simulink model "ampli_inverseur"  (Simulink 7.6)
settings: Solver=ode15s  StartTime=0.0  StopTime=0.001  FixedStep=0.01  RelTol=1e-5
InitFcn:
  | clc
StopFcn:
  | % lecture du fichier binaire
  | load inverseur.mat
  | 
  | % trace de la tension et du courant d’induit
  | plot(x(1,:),x(2,:),x(1,:),x(3,:))
  | title('Entrée/sortie - amplificateur inverseur - Composant ampli op')
  | grid
libraries: fl_lib x11, nesl_utility x4, MaLibrairieElectrical_lib x1

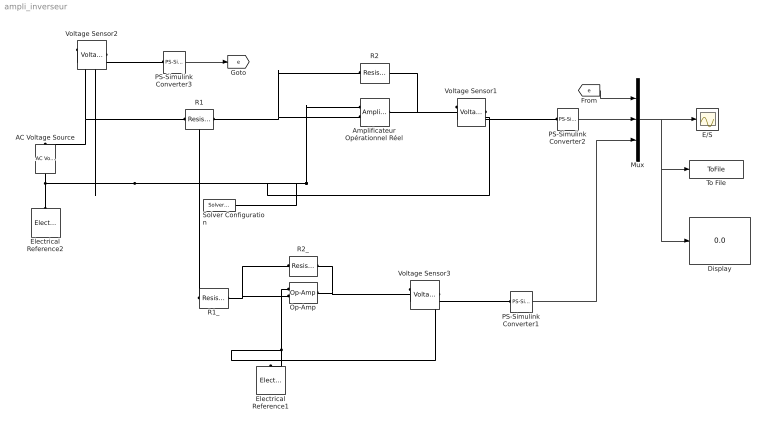
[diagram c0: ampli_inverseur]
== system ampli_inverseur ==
  AC Voltage Source : fl_lib/Electrical/Electrical Sources/AC Voltage Source  DialogController=NetworkEngine.DynNeDlgSource  SystemSampleTime=-1  amp=5 V  shift=0 rad  omega=2 kHz  i_Log=off  v_Log=off  LocalVarNames=|i|v  LocalVarDescs=|i|v  LocalVarLogging=[0 0]
  Amplificateur Opérationnel Réel : MaLibrairieElectrical_lib/Amplificateur Opérationnel Réel  DialogController=NetworkEngine.DynNeDlgSource  SystemSampleTime=-1  A=1e+6  Re=1e+6 Ohm  Rs=100 Ohm  Vsat=15 V  ie_Log=off  eps_Log=off  is_Log=off  vs_Log=off  LocalVarNames=|ie|eps|is|vs  LocalVarDescs=|ie|eps|is|vs  LocalVarLogging=[0 0 0 0]
  Display : Display
  E/S : Scope
  Electrical Reference1 : fl_lib/Electrical/Electrical Elements/Electrical Reference  DialogController=NetworkEngine.DynNeDlgSource  SystemSampleTime=-1  i_Log=off  LocalVarNames=|i  LocalVarDescs=|i  LocalVarLogging=0
  Electrical Reference2 : fl_lib/Electrical/Electrical Elements/Electrical Reference  DialogController=NetworkEngine.DynNeDlgSource  SystemSampleTime=-1  i_Log=off  LocalVarNames=|i  LocalVarDescs=|i  LocalVarLogging=0
  Mux : Mux  Inputs=3
  Op-Amp : fl_lib/Electrical/Electrical Elements/Op-Amp  DialogController=NetworkEngine.DynNeDlgSource  SystemSampleTime=-1  i1_Log=off  v1_Log=off  outI_Log=off  LocalVarNames=|i1|v1|outI  LocalVarDescs=|i1|v1|outI  LocalVarLogging=[0 0 0]
  PS-Simulink Converter1 : nesl_utility/PS-Simulink Converter  DialogController=NetworkEngine.DynNeUtilDlgSource  SystemSampleTime=-1  PhysicalDomain=network_engine_domain  LeftPortType=input  RightPortType=output  SubClassName=ps_output  Unit=1  AffineConversion=off
  PS-Simulink Converter2 : nesl_utility/PS-Simulink Converter  DialogController=NetworkEngine.DynNeUtilDlgSource  SystemSampleTime=-1  PhysicalDomain=network_engine_domain  LeftPortType=input  RightPortType=output  SubClassName=ps_output  Unit=1  AffineConversion=off
  PS-Simulink Converter3 : nesl_utility/PS-Simulink Converter  DialogController=NetworkEngine.DynNeUtilDlgSource  SystemSampleTime=-1  PhysicalDomain=network_engine_domain  LeftPortType=input  RightPortType=output  SubClassName=ps_output  Unit=1  AffineConversion=off
  R1 : fl_lib/Electrical/Electrical Elements/Resistor  DialogController=NetworkEngine.DynNeDlgSource  SystemSampleTime=-1  R=47 kOhm  i_Log=off  v_Log=off  LocalVarNames=|i|v  LocalVarDescs=|i|v  LocalVarLogging=[0 0]
  R1_ : fl_lib/Electrical/Electrical Elements/Resistor  DialogController=NetworkEngine.DynNeDlgSource  SystemSampleTime=-1  R=47 kOhm  i_Log=off  v_Log=off  LocalVarNames=|i|v  LocalVarDescs=|i|v  LocalVarLogging=[0 0]
  R2 : fl_lib/Electrical/Electrical Elements/Resistor  DialogController=NetworkEngine.DynNeDlgSource  SystemSampleTime=-1  R=100 kOhm  i_Log=off  v_Log=off  LocalVarNames=|i|v  LocalVarDescs=|i|v  LocalVarLogging=[0 0]
  R2_ : fl_lib/Electrical/Electrical Elements/Resistor  DialogController=NetworkEngine.DynNeDlgSource  SystemSampleTime=-1  R=100 kOhm  i_Log=off  v_Log=off  LocalVarNames=|i|v  LocalVarDescs=|i|v  LocalVarLogging=[0 0]
  Solver Configuration : nesl_utility/Solver Configuration  DialogController=NetworkEngine.DynNeUtilDlgSource  SystemSampleTime=-1  PhysicalDomain=network_engine_domain  LeftPortType=input  RightPortType=generic  SubClassName=solver  Accelerate=off  Profile=off  ResidualTolerance=1e-9  MaxNonlinIter=3  MaxModeIter=2  DoFixedCost=off  UseLocalSampling=off  DoDC=off  LinearAlgebra=Sparse  LocalSolverSampleTime=.001  LocalSolverChoice=NE_BACKWARD_EULER_ADVANCER  UseLocalSolver=off
  To File : ToFile  Filename=inverseur  MatrixName=x
  Voltage Sensor1 : fl_lib/Electrical/Electrical Sensors/Voltage Sensor  DialogController=NetworkEngine.DynNeDlgSource  SystemSampleTime=-1  i1_Log=off  v1_Log=off  LocalVarNames=|i1|v1  LocalVarDescs=|i1|v1  LocalVarLogging=[0 0]
  Voltage Sensor2 : fl_lib/Electrical/Electrical Sensors/Voltage Sensor  DialogController=NetworkEngine.DynNeDlgSource  SystemSampleTime=-1  i1_Log=off  v1_Log=off  LocalVarNames=|i1|v1  LocalVarDescs=|i1|v1  LocalVarLogging=[0 0]
  Voltage Sensor3 : fl_lib/Electrical/Electrical Sensors/Voltage Sensor  DialogController=NetworkEngine.DynNeDlgSource  SystemSampleTime=-1  i1_Log=off  v1_Log=off  LocalVarNames=|i1|v1  LocalVarDescs=|i1|v1  LocalVarLogging=[0 0]
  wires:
  PS-Simulink Converter2/1 -> Mux/2
  PS-Simulink Converter3/1 -> [e]
  [e] -> Mux/1
  Mux/1 -> E/S/1, To File/1, Display/1
  PS-Simulink Converter1/1 -> Mux/3
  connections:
  Voltage Sensor1/LConn1 -- R2/RConn1 -- Amplificateur Opérationnel Réel/RConn1
  Amplificateur Opérationnel Réel/LConn2 -- R1/RConn1 -- R2/LConn1
  Voltage Sensor2/LConn1 -- R1/LConn1 -- R1_/LConn1 -- AC Voltage Source/LConn1
  Voltage Sensor1/RConn1 -- PS-Simulink Converter2/LConn1
  Voltage Sensor2/RConn1 -- PS-Simulink Converter3/LConn1
  Voltage Sensor1/RConn2 -- AC Voltage Source/RConn1 -- Electrical Reference2/LConn1 -- Voltage Sensor2/RConn2 -- Amplificateur Opérationnel Réel/LConn1 -- Solver Configuration/RConn1
  R1_/RConn1 -- Op-Amp/LConn2 -- R2_/LConn1
  Op-Amp/LConn1 -- Electrical Reference1/LConn1 -- Voltage Sensor3/RConn2
  R2_/RConn1 -- Op-Amp/RConn1 -- Voltage Sensor3/LConn1
  Voltage Sensor3/RConn1 -- PS-Simulink Converter1/LConn1
